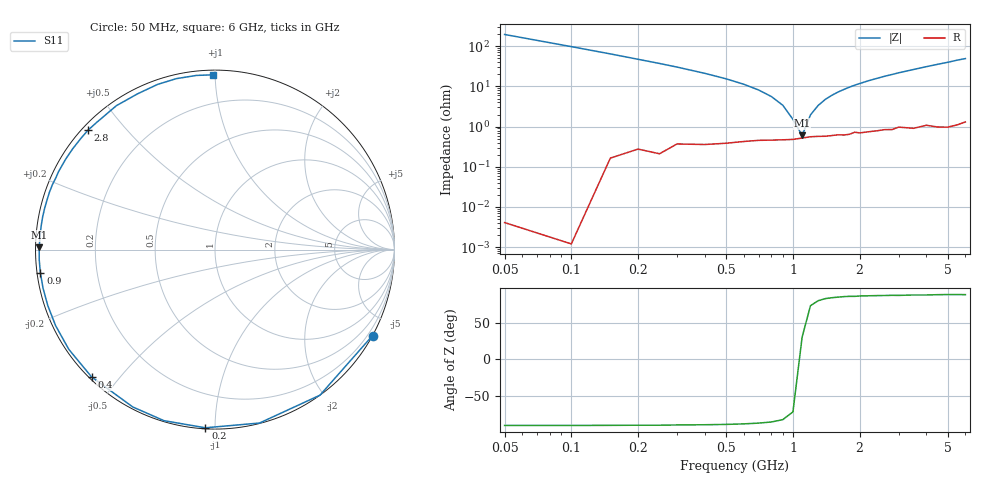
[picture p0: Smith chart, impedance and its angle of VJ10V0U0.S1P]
! Infineon Technologies  Discrete & RF Semiconductors
! BB 914
! Si Tuning Diode in SOT23
! VR = 10 V
! S-Parameters:  July  1999
# GHz  S  MA  R  50
!  f  S11
! GHz  MAG  ANG
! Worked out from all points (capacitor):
!   34 points, 50 MHz to 6 GHz, reference 50 ohm
!   read as one part to ground: C = 16.1 pF near 50 MHz
!   lowest |Z| = 603 mohm at 1.1 GHz (marker M1)
!   series resonance near 1.083 GHz, so ESL is about 1.3 nH
!   S11 on the Smith chart (normalised r, x): 50 MHz: 0.00, -3.92; 200 MHz: 0.01, -0.95; 400 MHz: 0.01, -0.42; 900 MHz: 0.01, -0.07; 2.8 GHz: 0.02, +0.40; 6 GHz: 0.03, +0.99
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0.05  1 -28.6
0.1  1 -54.2
0.15  0.9975 -75.6
0.2  0.9942 -93.1
0.25  0.9946 -106.6
0.3  0.9892 -117.6
0.4  0.9879 -134.1
0.5  0.986 -145.7
0.6  0.9839 -154.5
0.7  0.9824 -161.5
0.8  0.9819 -167.3
0.9  0.9815 -172.3
1.1  0.9794 179.3
1.2  0.9779 175.7
1.4  0.9775 169.2
1.6  0.9758 163.5
1.8  0.9754 158.3
2  0.9739 153.5
2.2  0.9727 148.9
2.4  0.9717 144.7
2.8  0.9712 136.8
3  0.9679 132.9
3.5  0.972 124.4
4  0.9693 116.4
4.5  0.9744 109.2
5  0.9766 102.8
5.5  0.9759 96.1
6  0.9738 90.8
